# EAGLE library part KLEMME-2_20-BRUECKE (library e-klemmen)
Klemme 20-pol. mit Brückenhinweis
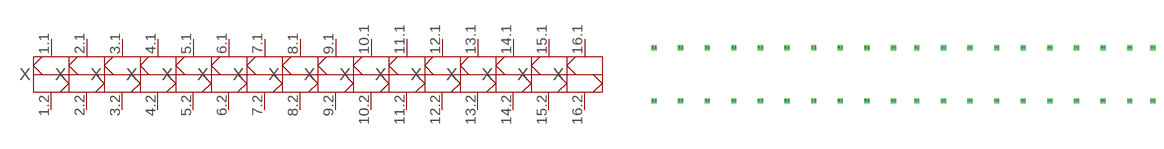
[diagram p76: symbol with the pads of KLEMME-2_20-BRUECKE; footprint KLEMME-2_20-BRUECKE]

Designator prefix X; gates 1=KLEMME-2_1-BRUECKE 2=KLEMME-2_2-BRUECKE 3=KLEMME-2_3-BRUECKE 4=KLEMME-2_4-BRUECKE 5=KLEMME-2_5-BRUECKE 6=KLEMME-2_6-BRUECKE 7=KLEMME-2_7-BRUECKE 8=KLEMME-2_8-BRUECKE 9=KLEMME-2_9-BRUECKE 10=KLEMME-2_10-BRUECKE 11=KLEMME-2_11-BRUECKE 12=KLEMME-2_12-BRUECKE 13=KLEMME-2_13-BRUECKE 14=KLEMME-2_14-BRUECKE 15=KLEMME-2_15-BRUECKE 16=KLEMME-2_16-BRUECKE 17=KLEMME-2_17-BRUECKE 18=KLEMME-2_18-BRUECKE 19=KLEMME-2_19-BRUECKE 20=KLEMME-2_20-BRUECKE

## KLEMME-2_20-BRUECKE  [KLEMME-2_20-BRUECKE]
1.1  1:1  pas
1.2  1:2  pas
2.1  2:1  pas
2.2  2:2  pas
3.1  3:1  pas
3.2  3:2  pas
4.1  4:1  pas
4.2  4:2  pas
5.1  5:1  pas
5.2  5:2  pas
6.1  6:1  pas
6.2  6:2  pas
7.1  7:1  pas
7.2  7:2  pas
8.1  8:1  pas
8.2  8:2  pas
9.1  9:1  pas
9.2  9:2  pas
10.1  10:1  pas
10.2  10:2  pas
11.1  11:1  pas
11.2  11:2  pas
12.1  12:1  pas
12.2  12:2  pas
13.1  13:1  pas
13.2  13:2  pas
14.1  14:1  pas
14.2  14:2  pas
15.1  15:1  pas
15.2  15:2  pas
16.1  16:1  pas
16.2  16:2  pas
17.1  17:1  pas
17.2  17:2  pas
18.1  18:1  pas
18.2  18:2  pas
19.1  19:1  pas
19.2  19:2  pas
20.1  20:1  pas
20.2  20:2  pas

## Footprint KLEMME-2_20-BRUECKE (pad centres in mm)
Dummy
drill 0.5 pad 1 square: 1.1 0,5.08; 1.2 0,-5.08; 2.1 5.08,5.08; 2.2 5.08,-5.08; 3.1 10.16,5.08; 3.2 10.16,-5.08; 4.1 15.24,5.08; 4.2 15.24,-5.08; 5.1 20.32,5.08; 5.2 20.32,-5.08; 6.1 25.4,5.08; 6.2 25.4,-5.08; 7.1 30.48,5.08; 7.2 30.48,-5.08; 8.1 35.56,5.08; 8.2 35.56,-5.08; 9.1 40.64,5.08; 9.2 40.64,-5.08; 10.1 45.72,5.08; 10.2 45.72,-5.08; 11.1 50.165,5.08; 11.2 50.165,-5.08; 12.1 55.245,5.08; 12.2 55.245,-5.08; 13.1 60.325,5.08; 13.2 60.325,-5.08; 14.1 65.405,5.08; 14.2 65.405,-5.08; 15.1 70.485,5.08; 15.2 70.485,-5.08; 16.1 75.565,5.08; 16.2 75.565,-5.08; 17.1 80.645,5.08; 17.2 80.645,-5.08; 18.1 85.725,5.08; 18.2 85.725,-5.08; 19.1 90.805,5.08; 19.2 90.805,-5.08; 20.1 95.25,5.08; 20.2 95.25,-5.08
